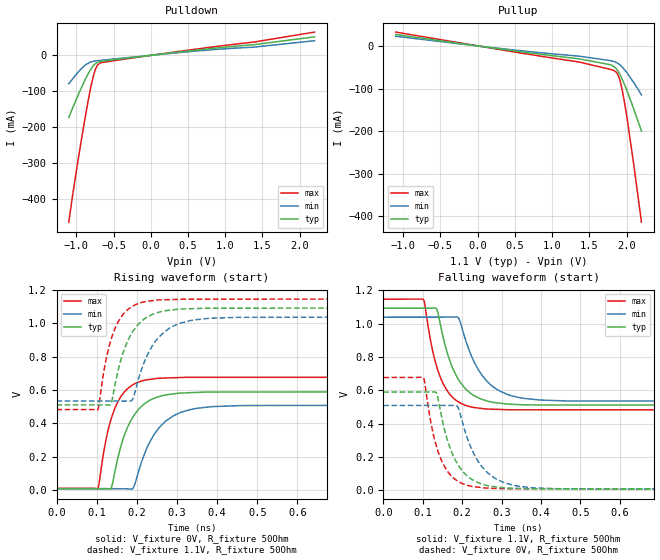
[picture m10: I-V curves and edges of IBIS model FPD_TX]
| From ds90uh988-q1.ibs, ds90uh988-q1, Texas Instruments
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[Model]   FPD_TX
Model_type   Output
Polarity   Non-Inverting
Vmeas = 0.55
Vref = 0.55
Cref = 0pF
Rref = 50
|   typ   min   max
C_comp   0.666pF   0.801pF   0.529pF
[Voltage Range]   1.1   1.045   1.155
[Temperature Range]   27   105   -40
[Pullup Reference]   1.1   1.045   1.155
[Pulldown Reference]   -0   -0   0
[Power Clamp Reference]   1.1   1.045   1.155
[GND Clamp Reference]   0   0   0
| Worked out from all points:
|   slope of the pulldown table from 0 to 0.165 V, typ, clamps not added: 41.2 ohm
|   slope of the pullup table from 0 to 0.165 V, typ, clamps not added: 41.4 ohm
|   falling waveform, V_fixture 1.1V, R_fixture 50Ohm: 20-80 % time 55.7ps typ, 67.5ps min, 45.8ps max; typ from 1.09 V to 0.511 V
|   rising waveform, V_fixture 0V, R_fixture 50Ohm: 20-80 % time 54.1ps typ, 65.8ps min, 44.1ps max; typ from 0.008 V to 0.589 V
|   rising waveform, V_fixture 1.1V, R_fixture 50Ohm: 20-80 % time 52.2ps typ, 62.5ps min, 42.9ps max; typ from 0.51 V to 1.09 V
|   falling waveform, V_fixture 0V, R_fixture 50Ohm: 20-80 % time 53.1ps typ, 63.1ps min, 44.1ps max; typ from 0.589 V to 0.008 V
[Pulldown]
|   Voltage   I(typ)   I(min)   I(max)
-1.1V     -172.7mA   -79.29mA   -464.7mA
-1.057V   -151.1mA   -67.81mA   -401.7mA
-977.9mV  -112.4mA   -47.86mA   -295.1mA
-882.2mV  -68.71mA   -28.03mA   -175.4mA
-832.7mV  -48.69mA   -21.31mA   -118.4mA
-796.4mV  -36.19mA   -18.32mA   -80.92mA
-756.8mV  -25.96mA   -16.43mA   -47.95mA
-707.3mV  -19.21mA   -14.98mA   -25.83mA
-667.7mV  -16.99mA   -14.07mA   -20.74mA
-275mV    -7.081mA   -5.967mA   -8.537mA
1.378V    29.2mA     22.4mA     36.34mA
2.2V      51.14mA    40.28mA    64.35mA
[Pullup]
|   Voltage   I(typ)   I(min)   I(max)
-1.1V     27.11mA    22.98mA    32.86mA
418mV     -9.597mA   -7.911mA   -11.77mA
1.385V    -30.87mA   -24.34mA   -38.46mA
1.774V    -43.69mA   -34.03mA   -54.61mA
1.824V    -47.31mA   -36.05mA   -57.31mA
1.863V    -53.64mA   -38.75mA   -62.04mA
1.896V    -62.26mA   -42.33mA   -72.73mA
1.923V    -71.04mA   -46.19mA   -88.58mA
1.972V    -90.53mA   -55.53mA   -132.8mA
2.009V    -106.4mA   -63.66mA   -172.2mA
2.098V    -148.5mA   -86.29mA   -280.1mA
2.2V      -199.9mA   -114.8mA   -414.6mA
[Ramp]
R_load = 50
|   typ   min   max
dV/dt_r   0.348562/5.38544e-11   0.300857/6.57676e-11   0.400265/4.38544e-11
dV/dt_f   0.348746/5.54814e-11   0.302286/6.74803e-11   0.398008/4.57236e-11
[Falling Waveform]
V_fixture = 1.1V
V_fixture_min = 1.045V
V_fixture_max = 1.155V
R_fixture = 50Ohm
C_fixture = 0F
|   Time   V(typ)   V(min)   V(max)
0s        1.092V     1.038V     1.146V
101.6ps   1.092V     1.038V     1.145V
134ps     1.092V     1.038V     752.8mV
164.1ps   809.5mV    1.039V     590mV
190.8ps   663.6mV    1.033V     530.3mV
217.1ps   589.6mV    843.1mV    503.4mV
243.4ps   551.7mV    714.5mV    492.8mV
271.7ps   530.7mV    634.4mV    487mV
349.9ps   513.6mV    553.9mV    483.2mV
1ns       510.8mV    534.2mV    482.3mV
[Rising Waveform]
V_fixture = 0V
V_fixture_min = 0V
V_fixture_max = 0V
R_fixture = 50Ohm
C_fixture = 0F
|   Time   V(typ)   V(min)   V(max)
0s        7.778mV    6.673mV    9.15mV
102.6ps   7.913mV    6.784mV    8.569mV
120.8ps   7.937mV    6.803mV    271.3mV
134.8ps   7.391mV    6.819mV    415.9mV
161.9ps   275.7mV    6.848mV    565.9mV
188.8ps   431.9mV    6.257mV    629.3mV
212.3ps   502.8mV    171.6mV    654mV
261.1ps   564.5mV    388.3mV    670.8mV
343.2ps   584.6mV    487.2mV    675.5mV
1ns       588.7mV    508.1mV    676.3mV
[Rising Waveform]
V_fixture = 1.1V
V_fixture_min = 1.045V
V_fixture_max = 1.155V
R_fixture = 50Ohm
C_fixture = 0F
|   Time   V(typ)   V(min)   V(max)
0s        510.4mV    533.6mV    482.1mV
102.8ps   510.5mV    533.3mV    481.7mV
119.7ps   510.5mV    533.2mV    736.1mV
134.4ps   511.2mV    533.1mV    891.5mV
160.1ps   778.3mV    533mV      1.035V
186.4ps   936.3mV    534.9mV    1.098V
212.3ps   1.014V     726.3mV    1.125V
265.5ps   1.073V     942.6mV    1.141V
343.2ps   1.088V     1.021V     1.145V
1ns       1.092V     1.037V     1.146V
[Falling Waveform]
|Gnd
V_fixture = 0V
V_fixture_min = 0V
V_fixture_max = 0V
R_fixture = 50Ohm
C_fixture = 0F
|   Time   V(typ)   V(min)   V(max)
0s        589.1mV    508.7mV    676.4mV
101.6ps   589.7mV    509mV      675.5mV
133.5ps   587.9mV    509.1mV    274.1mV
161.9ps   306.6mV    509.1mV    117mV
186.4ps   165.3mV    506.9mV    59.25mV
212.3ps   87.98mV    318.2mV    31.03mV
236ps     51.05mV    191.5mV    20.65mV
265.5ps   27.9mV     103.4mV    13.44mV
343.2ps   11.87mV    24.79mV    10.04mV
1ns       8.17mV     7.282mV    9.319mV
